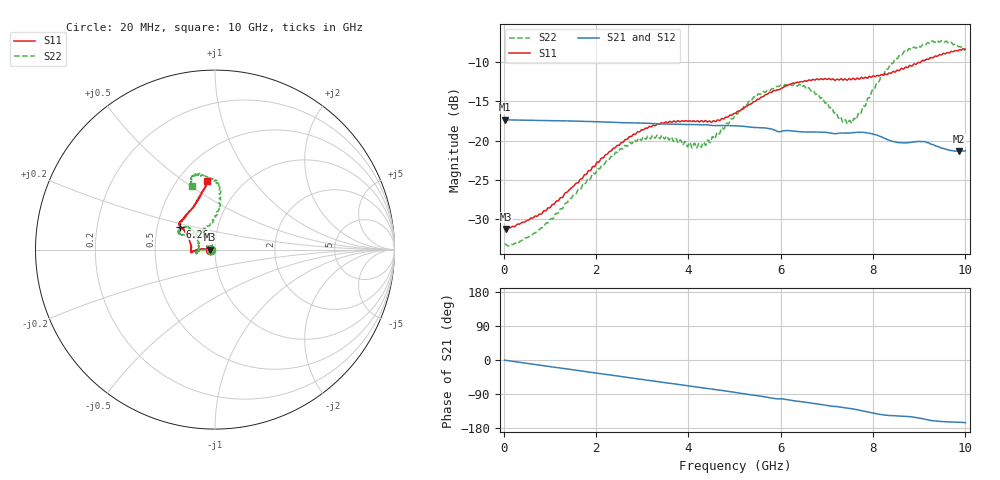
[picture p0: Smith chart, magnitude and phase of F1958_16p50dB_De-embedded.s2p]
! Integrated Device Technology
! Corporate Headquarters
! 6024 Silver Creek Valley Road
! San Jose, CA 95138  USA
! Phone:  1-408-284-8200
! Toll Free:  1-800-223-1366
! Webpage:  http://www.idt.com/
! Timing and RF Division
! 515 Groton Road, Suite 102
! Westford, MA 01886-6024
! Device:  F1958
! Description: 7-bit 0.25 dB Digital Step Attenuator
! Frequency:  0.001 -  6.000 GHz
! Package:  4x4 mm Thin QFN Plastic Package: 24 pin
! Ports:  2 RF, 12 DC
!  Pin  1  = D0
!  Pin  2  = VDD
!  Pin  3  = VMODE
!  Pin  4  = GND
!  Pin  5  = RF1  =  Port 1
!  Pin  6  = GND
!  Pin  7  = GND
!  Pin  8  = GND
!  Pin  9  = GND
!  Pin 10  = GND
!  Pin 11  = GND
!  Pin 12  = GND
!  Pin 13  = GND
!  Pin 14  = RF2  =  Port 2
!  Pin 15  = GND
!  Pin 16  = LE
!  Pin 17  = CLK
!  Pin 18  = DATA
!  Pin 19  = D6
!  Pin 20  = D5
!  Pin 21  = D4
!  Pin 22  = D3
!  Pin 23  = D2
!  Pin 24  = D1
! State:  66
! Atten State:  16.50 dB
! Voltage:  +3.30 Volts
! Current:  0.259 mA
! Data:  The device was measured on a F1958 evaluation board which has
!  individual transmission lines to the RF pins.  Data was collected
!  using a calibrated network analyzer.  The evaluation board was
!  de-embedded using Automatic Fixture Removal (AFR).
!  The reference plane is the edge of the package pin.
! Misc:
!  Action Tracker AT0419
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# GHz S dB R 50
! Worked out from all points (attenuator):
!   500 points, 20 MHz to 10 GHz, reference 50 ohm
!   highest |S21| = -17.33 dB at 20 MHz (marker M1); lowest = -21.4 dB at 9.86 GHz (marker M2)
!   lowest |S11| = -31.3 dB at 40 MHz (marker M3), VSWR 1.06, Z = 47.4 - j0.0726 ohm
!   |S11| at or under -10 dB: start of sweep to 9.027 GHz
!   |S22| runs from -33.5 to -7.2 dB; largest |S21 - S12| = 0.00052
!   S11 on the Smith chart (normalised r, x): 20 MHz: 0.95, -0.00; 6.26 GHz: 0.66, +0.18; 10 GHz: 0.69, +0.62
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0.02  -31.29 -178.4  -17.33 -0.5  -17.33 -0.4  -33.28 -178.2
0.04  -31.31 -178.4  -17.34 -0.8  -17.33 -0.8  -33.23 -177.4
0.3  -30.68 177.5  -17.37 -5.3  -17.37 -5.3  -33.20 178.5
0.72  -29.68 177.4  -17.41 -12.5  -17.40 -12.5  -31.63 178.1
1.7  -24.85 177.2  -17.54 -29.2  -17.54 -29.2  -25.76 178.1
2.6  -20.12 -179.0  -17.70 -44.5  -17.68 -44.5  -20.85 -176.5
2.92  -18.88 -176.1  -17.75 -50.0  -17.74 -50.1  -19.71 -172.9
3.36  -17.92 -173.7  -17.86 -57.5  -17.86 -57.6  -19.58 -168.1
4.26  -17.54 -179.8  -17.96 -72.5  -17.98 -72.6  -20.71 169.8
4.52  -17.60 174.2  -18.08 -77.1  -18.09 -77.2  -19.48 155.0
5.02  -16.52 160.8  -18.10 -85.7  -18.12 -85.7  -16.60 140.4
5.54  -14.66 150.5  -18.35 -94.9  -18.36 -94.9  -14.05 141.6
6.26  -12.67 146.4  -18.77 -107.0  -18.79 -107.0  -12.96 152.5
6.68  -12.22 144.3  -18.90 -113.8  -18.92 -113.7  -13.65 155.1
7.32  -12.12 138.2  -19.04 -124.9  -19.05 -124.8  -17.26 135.0
7.5  -12.13 135.0  -19.03 -127.9  -19.03 -127.9  -17.42 117.4
7.7  -12.16 130.8  -18.94 -132.3  -18.94 -132.3  -16.48 100.5
8.34  -11.37 115.9  -19.93 -146.4  -19.93 -146.5  -10.71 83.8
8.68  -10.74 109.2  -20.29 -148.5  -20.31 -148.5  -8.56 88.0
9.26  -9.38 101.3  -20.47 -159.5  -20.45 -159.5  -7.40 100.5
9.86  -8.43 96.6  -21.37 -164.3  -21.40 -164.2  -8.00 109.2
10  -8.32 96.5  -21.29 -165.4  -21.32 -165.1  -8.49 109.9
